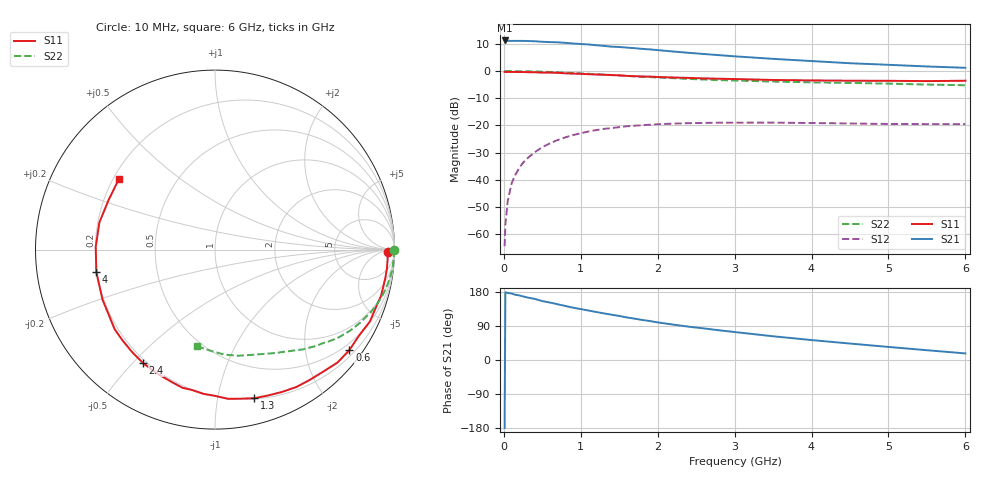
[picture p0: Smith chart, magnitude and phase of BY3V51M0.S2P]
! SIEMENS Small Signal Semiconductors
! BFY420
! Si NPN RF SIEGET Grounded Emitter Transistor in MICRO-X
! VCE = 3.5 V  IC = 1 mA
! Common Emitter S-Parameters:  October  1996
# GHz  S  MA  R  50
!  f  S11  S21  S12  S22
! GHz  MAG  ANG  MAG  ANG  MAG  ANG  MAG  ANG
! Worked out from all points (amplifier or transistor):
!   36 points, 10 MHz to 6 GHz, reference 50 ohm
!   highest |S21| = 11.3 dB at 10 MHz (marker M1)
!   |S21| within 3 dB of that: start of sweep to 1.762 GHz
!   unconditionally stable (mu >= 1): 4.479 GHz to end of sweep
!   at 250 MHz: K = 0.04, MSG = 22.4 dB, |S12| = -33.7 dB
!   at 1.4 GHz: K = 0.19, MSG = 15.0 dB, |S12| = -21.0 dB
!   at 6 GHz: K = 1.34, MAG = 6.9 dB, |S12| = -19.5 dB
!   S11 on the Smith chart (normalised r, x): 10 MHz: 50, -20; 600 MHz: 0.33, -2.97; 1.3 GHz: 0.21, -1.28; 2.4 GHz: 0.19, -0.54; 4 GHz: 0.20, -0.09; 6 GHz: 0.22, +0.31
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0.01  0.9659 -0.8  3.658 -179.4  0.0006 82.6  0.9989 -0.2
0.02  0.9602 -1.3  3.654 178.8  0.0015 76.7  0.9943 -0.6
0.05  0.9633 -3.0  3.605 177.0  0.004 83.4  0.9978 -1.4
0.1  0.9639 -6.4  3.592 175.6  0.0085 84.5  0.9964 -2.9
0.15  0.9619 -9.5  3.592 172.1  0.0124 82.8  0.9951 -4.3
0.3  0.954 -18.5  3.577 165.2  0.0244 78.2  0.9891 -8.5
0.4  0.9515 -24.9  3.537 161.3  0.032 74.9  0.9812 -11.3
0.5  0.935 -30.7  3.458 155.5  0.0397 71.3  0.9721 -14.1
0.6  0.935 -36.8  3.417 151.6  0.047 68.1  0.9615 -16.7
0.8  0.9091 -48.3  3.305 142.5  0.0603 60.7  0.935 -21.9
1.1  0.8759 -65.0  3.087 130.5  0.0774 51.7  0.8907 -29.0
1.3  0.8561 -75.3  2.909 123.1  0.0864 45.9  0.8603 -33.1
1.7  0.8062 -94.6  2.64 109.2  0.0988 36.3  0.7972 -40.7
2  0.7772 -107.7  2.429 99.2  0.1052 29.6  0.7619 -45.6
2.2  0.7616 -115.2  2.291 93.5  0.1079 25.7  0.7404 -48.7
2.4  0.7488 -122.4  2.168 88.0  0.11 22.7  0.7171 -51.5
3  0.7135 -141.6  1.868 73.8  0.1123 14.7  0.6696 -59.3
3.5  0.6859 -156.0  1.678 62.6  0.1126 9.8  0.6411 -65.1
4  0.6729 -169.3  1.528 52.6  0.1107 6.3  0.6199 -71.2
4.5  0.6647 178.7  1.394 43.4  0.1086 3.9  0.6054 -77.6
5.5  0.6541 155.0  1.215 25.8  0.1057 3.0  0.5651 -92.1
6  0.6638 143.9  1.149 17.4  0.1055 3.9  0.548 -100.4
